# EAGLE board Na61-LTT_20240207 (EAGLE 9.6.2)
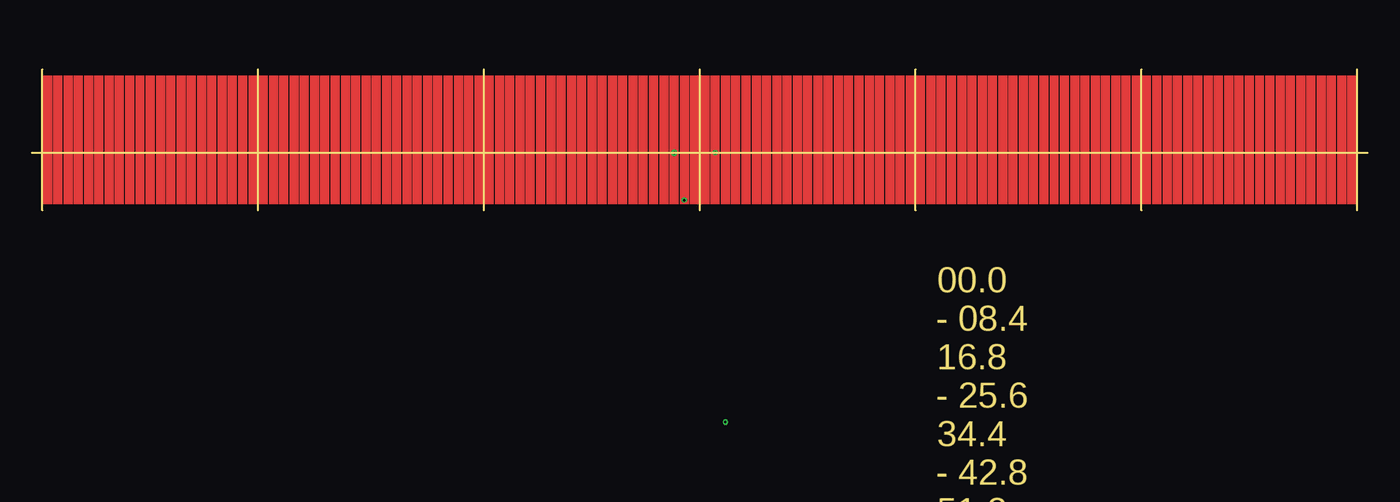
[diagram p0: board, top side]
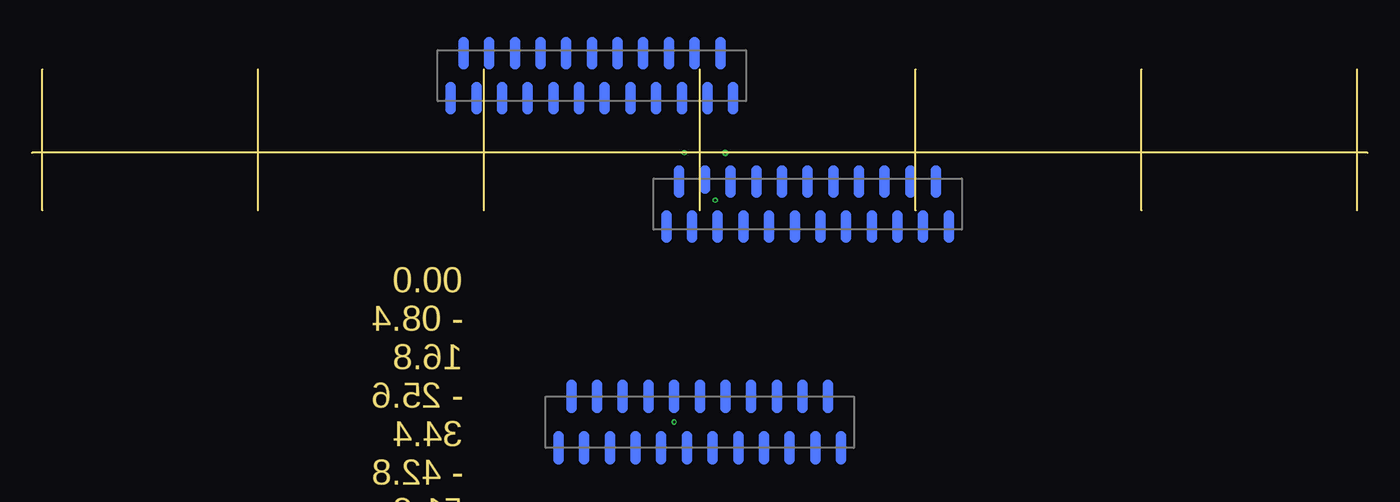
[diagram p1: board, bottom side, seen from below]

Size 104 x 11 mm. Coordinates in mm from the lower left corner, seen from the top.
Outline: 52,0 52,11
Outline: 35.2,0 35.2,11
Outline: 17.6,0 17.6,11
Outline: 0.8,0 0.8,11
Outline: 68.8,0 68.8,11
Outline: 86.4,0 86.4,11
Outline: 103.2,0 103.2,11
Outline: 0,4.5 104,4.5
Copper layers (1*16): Top 0.035mm / dielectric 1.5mm / Bottom 0.035mm
Design rules "default *": minimum track width 6mil, minimum drill 0.2mm, track to track 6mil, track to pad 6mil, pad to pad 6mil, via to via 6mil, smd to smd 6mil, copper to edge 40mil, drill to drill 6mil, minimum pad ring 8mil, minimum via ring 4mil, stop-mask expansion 4mil, vias tented up to drill 0mil, thermal gap 10mil

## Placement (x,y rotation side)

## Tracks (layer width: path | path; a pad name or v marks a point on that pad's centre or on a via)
S$1
  Bottom 0.8: 55,-17.6 55,-19.4
S$2
  Bottom 0.8: 54,-15.4 54,-13.6
S$3
  Bottom 0.8: 51,-17.6 51,-19.4
S$4
  Bottom 0.8: 48,-15.4 48,-13.6
S$5
  Bottom 0.8: 45,-17.6 45,-19.4
S$6
  Bottom 0.8: 44,-15.4 44,-13.6
S$7
  Bottom 0.8: 41,-17.6 41,-19.4
S$8
  Bottom 0.8: 42,-15.4 42,-13.6
S$9
  Bottom 0.8: 63,-17.6 63,-19.4
S$10
  Bottom 0.8: 62,-15.4 62,-13.6
S$11
  Bottom 0.8: 59,-17.6 59,-19.4
S$12
  Bottom 0.8: 58,-15.4 58,-13.6
S$13
  Bottom 0.8: 60,-15.4 60,-13.6
S$14
  Bottom 0.8: 61,-17.6 61,-19.4
S$15
  Bottom 0.8: 57,-17.6 57,-19.4
S$16
  Bottom 0.8: 56,-15.4 56,-13.6
S$17
  Bottom 0.8: 52,-15.4 52,-13.6
S$18
  Bottom 0.8: 53,-17.6 53,-19.4
S$19
  Bottom 0.8: 49,-17.6 49,-19.4
S$20
  Bottom 0.8: 50,-15.4 50,-13.6
S$21
  Bottom 0.8: 46,-15.4 46,-13.6
S$22
  Bottom 0.8: 47,-17.6 47,-19.4
S$23
  Bottom 0.8: 43,-17.6 43,-19.4
S$24
  Bottom 0.8: 61.4,9.6 61.4,7.9
S$25
  Bottom 0.8: 63.4,9.6 63.4,7.9
S$26
  Bottom 0.8: 60.4,11.4 60.4,13.1
S$27
  Bottom 0.8: 62.4,11.4 62.4,13.1
S$28
  Bottom 0.8: 57.4,9.6 57.4,7.9
S$29
  Bottom 0.8: 59.4,9.6 59.4,7.9
S$30
  Bottom 0.8: 58.4,11.4 58.4,13.1
S$31
  Bottom 0.8: 56.4,11.4 56.4,13.1
S$32
  Bottom 0.8: 55.4,9.6 55.4,7.9
S$33
  Bottom 0.8: 53.4,9.6 53.4,7.9
S$34
  Bottom 0.8: 54.4,11.4 54.4,13.1
S$35
  Bottom 0.8: 52.4,11.4 52.4,13.1
S$36
  Bottom 0.8: 51.4,9.6 51.4,7.9
S$37
  Bottom 0.8: 49.4,9.6 49.4,7.9
S$38
  Bottom 0.8: 50.4,11.4 50.4,13.1
S$39
  Bottom 0.8: 69.4,9.6 69.4,7.9
S$40
  Bottom 0.8: 71.4,9.6 71.4,7.9
S$41
  Bottom 0.8: 68.4,11.4 68.4,13.1
S$42
  Bottom 0.8: 70.4,11.4 70.4,13.1
S$43
  Bottom 0.8: 65.4,9.6 65.4,7.9
S$44
  Bottom 0.8: 67.4,9.6 67.4,7.9
S$45
  Bottom 0.8: 64.4,11.4 64.4,13.1
S$46
  Bottom 0.8: 66.4,11.4 66.4,13.1
S$47
  Bottom 0.8: 44.6,-0.4 44.6,-2.1
S$48
  Bottom 0.8: 46.6,-0.4 46.6,-2.1
S$49
  Bottom 0.8: 43.6,1.4 43.6,3.1
S$50
  Bottom 0.8: 45.6,1.4 45.6,3.1
S$51
  Bottom 0.8: 40.6,-0.4 40.6,-2.1
S$52
  Bottom 0.8: 42.6,-0.4 42.6,-2.1
S$53
  Bottom 0.8: 41.6,1.4 41.6,3.1
S$54
  Bottom 0.8: 39.6,1.4 39.6,3.1
S$55
  Bottom 0.8: 38.6,-0.4 38.6,-2.1
S$56
  Bottom 0.8: 36.6,-0.4 36.6,-2.1
S$57
  Bottom 0.8: 37.6,1.4 37.6,3.1
S$58
  Bottom 0.8: 35.6,1.4 35.6,3.1
S$59
  Bottom 0.8: 34.6,-0.4 34.6,-2.1
S$60
  Bottom 0.8: 32.6,-0.4 32.6,-2.1
S$61
  Bottom 0.8: 33.6,1.4 33.6,3.1
S$62
  Bottom 0.8: 52.6,-0.4 52.6,-2.1
S$63
  Bottom 0.8: 54.6,-0.4 54.6,-2.1
S$64
  Bottom 0.8: 51.6,1.7 51.6,3.1
S$65
  Bottom 0.8: 53.6,1.4 53.6,3.1
S$66
  Bottom 0.8: 48.6,-0.4 48.6,-2.1
S$67
  Bottom 0.8: 50.6,-0.4 50.6,-2.1
S$68
  Bottom 0.8: 47.6,1.4 47.6,3.1
S$69
  Bottom 0.8: 49.6,1.4 49.6,3.1
S$70  (via drill 0.2 pad 0.5)
  other vias: 50,4.5
S$71  (via drill 0.2)
  other vias: 54,-16.5
S$72  (via drill 0.2)
  other vias: 53.2,4.5
S$73  (via drill 0.2)
  other vias: 50.8,0.8
(copper drawn outside any net)
  shapes: Top area x128

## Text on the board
Dimension: 00.0 / - 08.4 / 16.8 / - 25.6 / 34.4 / - 42.8 / 51.2
ConnRoute: Pad: 0.8 x 8 / VIA: szélén szélére, belül pont középre / PadRaw távolság : 8mm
